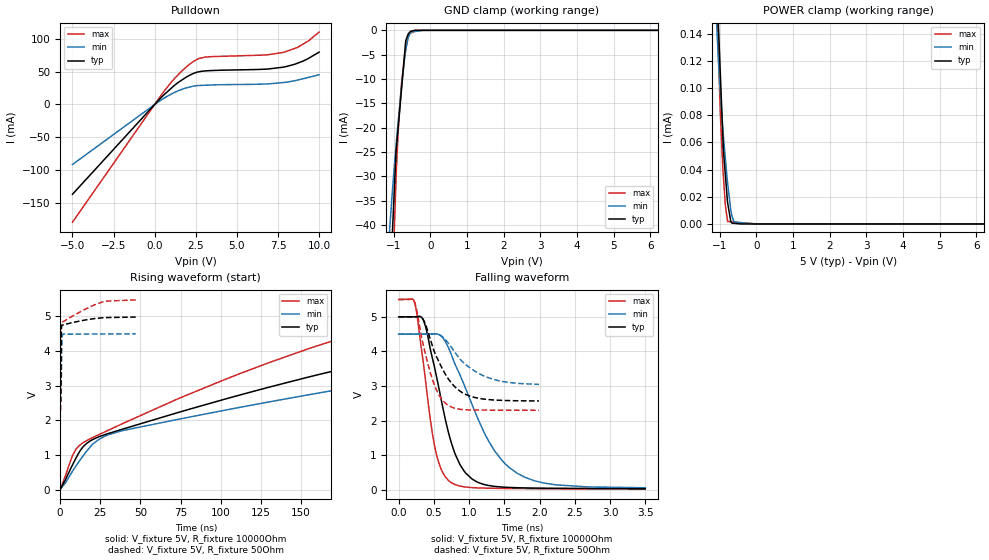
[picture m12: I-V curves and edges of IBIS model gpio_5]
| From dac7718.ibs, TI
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|   gpio_5 Model
[Model]   gpio_5
Model_type   I/O_open_drain
Polarity   Non-Inverting
Enable   Active-Low
Vinl = 0.8
Vinh = 3.8
Vmeas = 2.5
Vref = 5
Cref = 15pF
Rref = 10000
|   typ   min   max
|   (nom PVT)   (Fast PVT)   (slow PVT)
|C_comp from Frequency Method (F=50MHz)
|Average
|C_comp   3.407e-12   2.846e-12   3.888e-12
|OFF state: BUFFER IN HIGH IMPEDANCE
|C_comp   3.297e-12   2.719e-12   3.766e-12
|ON state : BUFFER OUTPUT TURNED LOW
C_comp   3.517e-12   2.973e-12   4.010e-12
|C_comp from LC Tank Method(L=1nH)
|Resonant Frequency(Hz)   3.08e9   3.25e9   2.950e9
|C_comp   2.673e-12   2.401e-12   2.914e-12
| Where nom  PVT is Nominal Process,  5V,  33C
|   Fast PVT is Strong Process,   5.5V,  -40C
|   Slow PVT is Weak Process,   4.5V,  113C
[Voltage Range]   5   4.5   5.5
[Temperature Range]   33   113   -40
[Pullup Reference]   5   4.5   5.5
[Pulldown Reference]   0   0   0
[Power Clamp Reference]   5   4.5   5.5
[GND Clamp Reference]   0   0   0
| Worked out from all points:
|   slope of the pulldown table from 0 to 0.75 V, typ, clamps not added: 39.7 ohm
|   GND clamp passes 1 mA (typ) near -0.61 V on its own axis
|   falling waveform, V_fixture 5V, R_fixture 10000Ohm: 20-80 % time 347ps typ, 625ps min, 224ps max; typ from 5 V to 0.036 V
|   rising waveform, V_fixture 5V, R_fixture 10000Ohm: 20-80 % time 215ns typ, 258ns min, 168ns max; typ from 0.018 V to 5 V
|   rising waveform, V_fixture 5V, R_fixture 50Ohm: 20-80 % time 248ps typ, 307ps min, 1.23ns max; typ from 2.55 V to 4.98 V
|   falling waveform, V_fixture 5V, R_fixture 50Ohm: 20-80 % time 337ps typ, 446ps min, 240ps max; typ from 5 V to 2.57 V
[Pulldown]
|   Voltage   I(typ)   I(min)   I(max)
-5V       -136.5mA   -91.21mA   -178.9mA
528mV     13.89mA    8.876mA    18.73mA
1.221V    29.43mA    18.44mA    39.85mA
2.007V    42.76mA    25.78mA    58.81mA
2.684V    49.65mA    28.82mA    69.89mA
3.08V     51.01mA    29.23mA    71.98mA
6.6V      53.49mA    31mA       75.06mA
7.854V    56.91mA    33.43mA    79.28mA
8.684V    62.67mA    37.04mA    86.67mA
9.345V    69.89mA    41.09mA    96.42mA
10V       79.54mA    45.11mA    110mA
[GND Clamp]
|   Voltage   I(typ)   I(min)   I(max)
-5V       -932.3mA   -650.1mA   -1.312A
-1.121V   -55.89mA   -42.13mA   -77.98mA
-1.095V   -51.55mA   -39.31mA   -70.39mA
-1.022V   -39.39mA   -31.72mA   -50.85mA
-1.001V   -35.98mA   -29.82mA   -45.38mA
-935mV    -24.98mA   -23.68mA   -30.58mA
-863.5mV  -18.82mA   -17.8mA    -19.1mA
-792mV    -12.65mA   -12.06mA   -11.42mA
-670mV    -2.134mA   -4.049mA   -3.859mA
-588.5mV  -608.4uA   -1.296mA   -914.7uA
-540mV    -206.6uA   -390.4uA   -620.7uA
10V       0A         0A         0A
[POWER Clamp]
|   Voltage   I(typ)   I(min)   I(max)
-5V       5.102mA    4.13mA     6.399mA
-1.095V   184.4uA    151.9uA    188.9uA
-1.034V   143.2uA    117.9uA    122.1uA
-984.5mV  109.5uA    96.74uA    80.41uA
-924mV    68.33uA    72.3uA     44.6uA
-905mV    55.39uA    65.72uA    35.75uA
-847mV    35.41uA    47.68uA    13.22uA
-790mV    16.1uA     30.77uA    2.458uA
-670mV    627.3nA    5.868uA    1.531uA
-616.5mV  484.6nA    1.651uA    1.408uA
0V        0A         0A         0A
10V       0A         0A         0A
[Ramp]
R_load = 10000
|   typ   min   max
dV/dt_r   2.98934/2.14774e-07   2.68492/2.59082e-07   3.29123/1.67894e-07
dV/dt_f   2.98935/3.49073e-10   2.68523/6.34413e-10   3.29123/2.26961e-10
[Falling Waveform]
V_fixture = 5V
V_fixture_min = 4.5V
V_fixture_max = 5.5V
R_fixture = 10000Ohm
|   Time   V(typ)   V(min)   V(max)
0s        5V         4.5V       5.5V
228ps     5.001V     4.5V       5.402V
354ps     4.889V     4.5V       3.617V
526ps     3.382V     4.51V      1.117V
722ps     1.54V      4.034V     246mV
868ps     740mV      3.329V     111.6mV
1.04ns    316.3mV    2.473V     65.84mV
1.35ns    104.6mV    1.163V     46.76mV
1.678ns   62.53mV    485.6mV    39.14mV
3.498ns   36.18mV    61.34mV    21.2mV
[Rising Waveform]
V_fixture = 5V
V_fixture_min = 4.5V
V_fixture_max = 5.5V
R_fixture = 10000Ohm
|   Time   V(typ)   V(min)   V(max)
0s        17.75mV    24.61mV    14.62mV
10.05ns   926.9mV    696.5mV    1.178V
16.53ns   1.335V     1.112V     1.415V
30.05ns   1.621V     1.584V     1.715V
153.8ns   3.239V     2.73V      4.054V
209.2ns   3.84V      3.164V     4.83V
246.6ns   4.195V     3.431V     5.185V
328.3ns   4.75V      3.937V     5.437V
420.5ns   4.934V     4.307V     5.487V
770.3ns   4.999V     4.489V     5.5V
[Rising Waveform]
V_fixture = 5V
V_fixture_min = 4.5V
V_fixture_max = 5.5V
R_fixture = 50Ohm
|   Time   V(typ)   V(min)   V(max)
0s        2.554V     3.029V     2.289V
280ps     2.548V     3.029V     2.357V
410ps     2.643V     3.026V     3.701V
530ps     3.342V     3.019V     4.608V
660ps     4.234V     3.079V     4.786V
790ps     4.595V     3.37V      4.816V
1.15ns    4.741V     4.298V     4.824V
1.78ns    4.755V     4.489V     4.844V
26.21ns   4.959V     4.492V     5.413V
47.07ns   4.981V     4.496V     5.475V
[Falling Waveform]
V_fixture = 5V
V_fixture_min = 4.5V
V_fixture_max = 5.5V
R_fixture = 50Ohm
|   Time   V(typ)   V(min)   V(max)
0s        5V         4.5V       5.5V
220ps     5.001V     4.5V       5.453V
260ps     5.004V     4.5V       5.147V
340ps     4.951V     4.5V       4.27V
460ps     4.282V     4.503V     3.314V
560ps     3.751V     4.495V     2.792V
680ps     3.284V     4.302V     2.477V
890ps     2.827V     3.736V     2.324V
1.19ns    2.629V     3.31V      2.305V
1.99ns    2.57V      3.05V      2.3V
